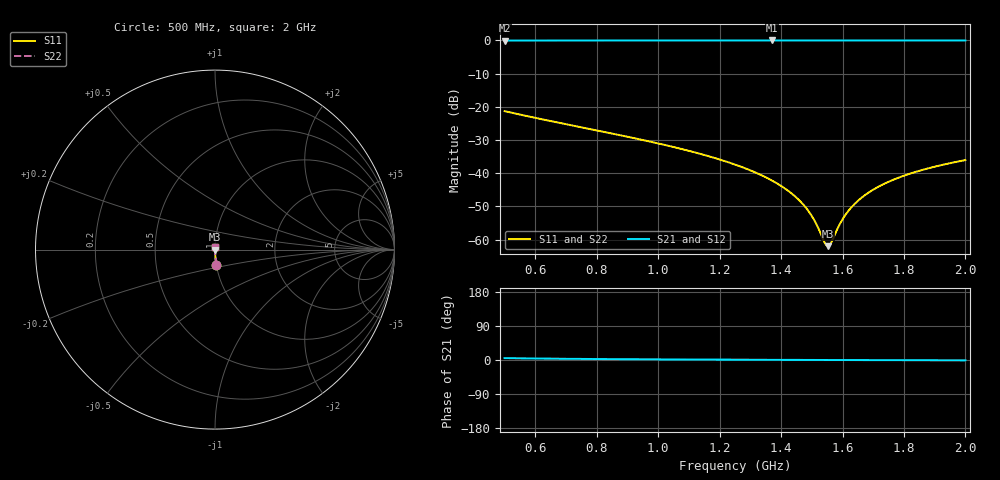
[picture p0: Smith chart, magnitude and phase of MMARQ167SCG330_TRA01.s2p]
! MMARQ167SCG330_TRA01  S-PARAMETER MODEL  ( General Type )
! Model Generated by TAIYO YUDEN Corporation (http://www.ty-top.com)
! Version 1.0
! TAIYO YUDEN Control No. 160201
! Copyright(c) 2016 TAIYO YUDEN CO.,LTD. All Rights Reserved.
! Product Description (link to TY-COMPAS)
! https://ds.yuden.co.jp/TYCOMPAS/or/detail?pn=MMARQ167SCG330JTRA01&u=M
! Products Name : Multilayer Ceramic Capacitors
! Characteristics :
!  Capacitance : 33 pF , Rated Voltage : 250V , TCC : CG / C0G
!  Case Size : 1.6 x 0.8 / 0.063 x 0.031 [mm/inch] , Thickness : 0.7 / 0.028 [mm/inch]
!  (Conditions: Temperature = 25 degC , DC Bias Current/Voltage = 0A / 0V)
! External Node Assignments :
!  1  o---| |---o  2
! GND o---------o GND
! Frequency Range : 500MHz  -  2000MHz  [ 401 STEP ]
# MHz S RI R 50
! Freq[MHz].  S11 Real  S11 Imag  S21 Real  S21 Imag  S12 Real  S12 Imag  S22 Real  S22 Imag
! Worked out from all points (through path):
!   401 points, 500 MHz to 2 GHz, reference 50 ohm
!   highest |S21| = -0.01 dB at 1.37 GHz (marker M1); lowest = 0.0 dB at 500 MHz (marker M2)
!   lowest |S11| = -62.0 dB at 1.554 GHz (marker M3), VSWR 1.00, Z = 50.1 + j0.00422 ohm
!   |S11| at or under -10 dB: start of sweep to end of sweep
!   |S22| runs from -62.0 to -21.3 dB; largest |S21 - S12| = 0
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500  0.00777 -0.0858  0.9922 0.0858  0.9922 0.0858  0.00777 -0.0858
751.25  0.00287 -0.0489  0.9971 0.0489  0.9971 0.0489  0.00287 -0.0489
1002.5  0.00137 -0.0279  0.9986 0.0279  0.9986 0.0279  0.00137 -0.0279
1141.25  0.00102 -0.0193  0.999 0.0193  0.999 0.0193  0.00102 -0.0193
1250  0.000873 -0.0135  0.9991 0.0135  0.9991 0.0135  0.000873 -0.0135
1313.75  0.000823 -0.0104  0.9992 0.0104  0.9992 0.0104  0.000823 -0.0104
1370  0.000796 -0.00774  0.9992 0.00774  0.9992 0.00774  0.000796 -0.00774
1411.25  0.000785 -0.0059  0.9992 0.0059  0.9992 0.0059  0.000785 -0.0059
1448.75  0.000781 -0.00427  0.9992 0.00427  0.9992 0.00427  0.000781 -0.00427
1478.75  0.000781 -0.00301  0.9992 0.00301  0.9992 0.00301  0.000781 -0.00301
1501.25  0.000784 -0.00208  0.9992 0.00208  0.9992 0.00208  0.000784 -0.00208
1516.25  0.000786 -0.00146  0.9992 0.00146  0.9992 0.00146  0.000786 -0.00146
1542.5  0.000792 -0.000406  0.9992 0.000406  0.9992 0.000406  0.000792 -0.000406
1553.75  0.000796 4.21e-05  0.9992 -4.21e-05  0.9992 -4.21e-05  0.000796 4.21e-05
1565  0.000799 0.000486  0.9992 -0.000486  0.9992 -0.000486  0.000799 0.000486
1587.5  0.000807 0.00137  0.9992 -0.00137  0.9992 -0.00137  0.000807 0.00137
1602.5  0.000814 0.00194  0.9992 -0.00194  0.9992 -0.00194  0.000814 0.00194
1636.25  0.00083 0.00323  0.9992 -0.00323  0.9992 -0.00323  0.00083 0.00323
1685  0.000858 0.00504  0.9991 -0.00504  0.9991 -0.00504  0.000858 0.00504
1752.5  0.000906 0.00747  0.9991 -0.00747  0.9991 -0.00747  0.000906 0.00747
1861.25  0.001 0.0112  0.999 -0.0112  0.999 -0.0112  0.001 0.0112
2000  0.00115 0.0157  0.9988 -0.0157  0.9988 -0.0157  0.00115 0.0157
